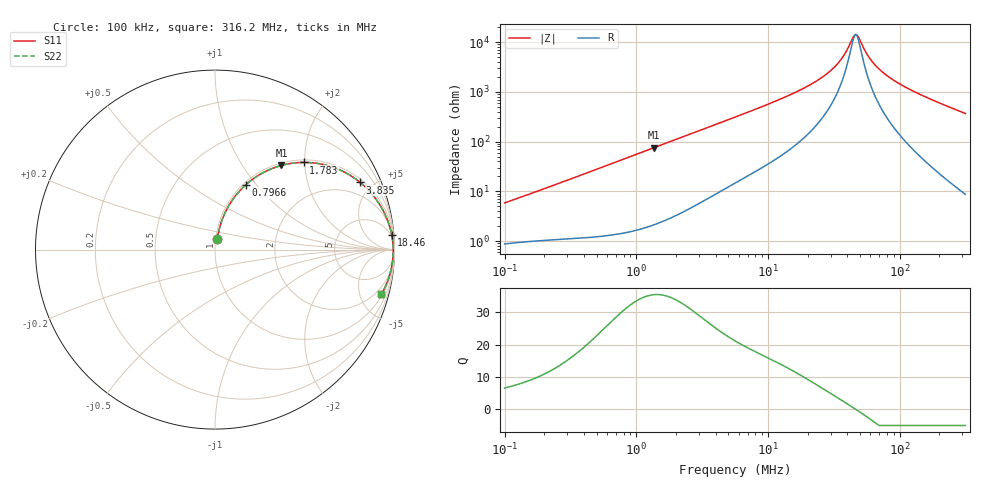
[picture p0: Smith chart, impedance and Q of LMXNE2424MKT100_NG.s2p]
! LMXNE2424MKT100_NG  S-PARAMETER MODEL  ( General Type )
! Model Generated by TAIYO YUDEN Corporation (http://www.ty-top.com)
! Version 1.0
! TAIYO YUDEN Control No. 191023NI43SB-FBB
! Copyright(c) 2019 TAIYO YUDEN CO.,LTD. All Rights Reserved.
! Product Description (link to TY-COMPAS)
! https://ds.yuden.co.jp/TYCOMPAS/or/detail?pn=LMXNE2424MKT100MNG&u=M
! Products Name : Inductors
! Characteristics :
!  Inductance : 10 uH , SRF(min) : 29 MHz , DC Resistance(max) : 0.72 Ohm
!  Rated Current : Saturation :810 mA , Temp Rise : 450 mA
!  Case Size : 2.4 x 2.4 / 0.094 x 0.094 [mm/inch] , Thickness : 1.2 / 0.047 [mm/inch]
!  (Conditions: Temperature = 25 degC , DC Bias Current/Voltage = 0A / 0V)
! External Node Assignments :
!  1  o---GGG---o  2
! GND o---------o GND
! Frequency Range : 0.1MHz  -  316.199832MHz  [ 402 STEP ]
# MHz S RI R 50
! Freq[MHz].  S11 Real  S11 Imag  S21 Real  S21 Imag  S12 Real  S12 Imag  S22 Real  S22 Imag
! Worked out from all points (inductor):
!   401 points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, 100 kHz to 316.2 MHz, reference 50 ohm
!   read as one part in series: L = 9.11 uH near 104.1 kHz
!   highest Q = 35.5 at 1.372 MHz (marker M1), where L = 8.82 uH
!   self-resonance near 45.71 MHz
!   S11 on the Smith chart (normalised r, x): 100 kHz: 1.02, +0.12; 796.6 kHz: 1.03, +0.88; 1.783 MHz: 1.06, +1.98; 3.835 MHz: 1.16, +4.23; 18.46 MHz: 3, +23; 316.2 MHz: 1.17, -7.35
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0.1  0.012 0.0567  0.988 -0.0567  0.988 -0.0567  0.012 0.0567
0.385695  0.0541 0.201  0.9459 -0.201  0.9459 -0.201  0.0541 0.201
0.7966  0.1716 0.3611  0.8284 -0.3611  0.8284 -0.3611  0.1716 0.3611
1.372422  0.3703 0.469  0.6297 -0.469  0.6297 -0.469  0.3703 0.469
1.487603  0.4074 0.4775  0.5926 -0.4775  0.5926 -0.4775  0.4074 0.4775
1.783349  0.4942 0.4858  0.5058 -0.4858  0.5058 -0.4858  0.4942 0.4858
3.834711  0.8086 0.3745  0.1914 -0.3745  0.1914 -0.3745  0.8086 0.3745
5.623165  0.8953 0.2834  0.1047 -0.2834  0.1047 -0.2834  0.8953 0.2834
11.15521  0.9663 0.1503  0.0337 -0.1503  0.0337 -0.1503  0.9663 0.1503
18.45972  0.9846 0.0835  0.0154 -0.0835  0.0154 -0.0835  0.9846 0.0835
21.68824  0.9876 0.0663  0.0124 -0.0663  0.0124 -0.0663  0.9876 0.0663
27.61997  0.9906 0.0433  0.0094 -0.0433  0.0094 -0.0433  0.9906 0.0433
33.11101  0.992 0.0275  0.00804 -0.0275  0.00804 -0.0275  0.992 0.0275
38.12604  0.9926 0.0159  0.00738 -0.0159  0.00738 -0.0159  0.9926 0.0159
44.79411  0.993 0.00294  0.00699 -0.00294  0.00699 -0.00294  0.993 0.00294
46.63594  0.993 -0.000279  0.00695 0.000279  0.00695 0.000279  0.993 -0.000279
48.5535  0.9931 -0.0035  0.00693 0.0035  0.00693 0.0035  0.9931 -0.0035
55.90748  0.993 -0.0149  0.00705 0.0149  0.00705 0.0149  0.993 -0.0149
61.83287  0.9927 -0.0232  0.0073 0.0232  0.0073 0.0232  0.9927 -0.0232
83.65039  0.9909 -0.0498  0.00908 0.0498  0.00908 0.0498  0.9909 -0.0498
141.2425  0.9819 -0.1077  0.0181 0.1077  0.0181 0.1077  0.9819 -0.1077
316.1998  0.926 -0.2501  0.074 0.2501  0.074 0.2501  0.926 -0.2501
